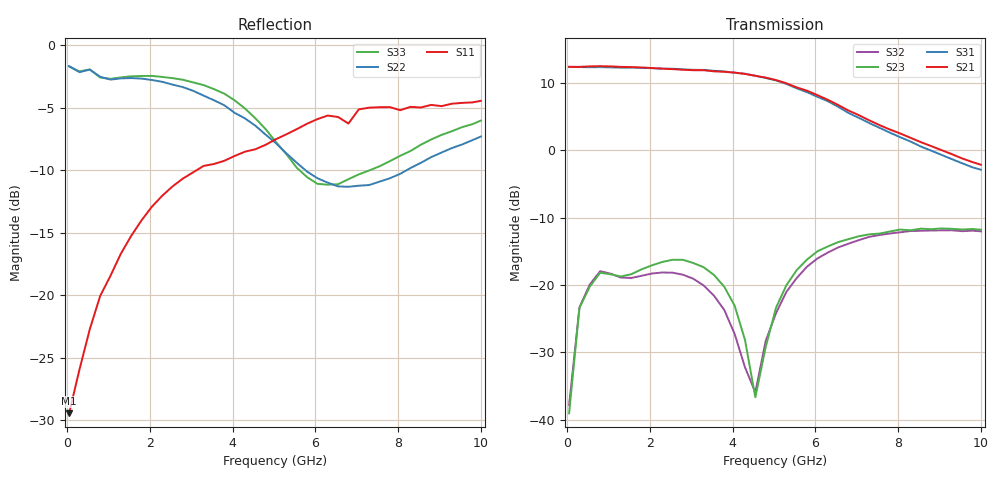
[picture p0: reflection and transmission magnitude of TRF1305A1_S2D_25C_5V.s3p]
! Created Tue Jun 24 15:00:24 2025
# hz S ma R 50
! 3 Port Network Data from SP1.SP block
! PORT[1] = INP
! PORT[2] = OUTM
! PORT[3] = OUTP
! freq  magS11  angS11  magS12  angS12  magS13  angS13
!  magS21  angS21
!  magS22  angS22  magS23  angS23
!  magS31  angS31  magS32  angS32
!  magS33  angS33
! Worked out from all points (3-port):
!   41 points, 50 MHz to 10 GHz, reference 50 ohm
!   strongest paths, dB at 50 MHz, 2.55 GHz, 5.05 GHz, 7.55 GHz, 10 GHz:
!     S21: 12.4, 12.0, 10.4, 3.7, -2.2
!     S31: 12.3, 12.1, 10.3, 3.3, -2.9
!     S23: -39.0, -16.2, -23.4, -12.4, -11.8
!     S32: -37.8, -18.2, -24.2, -12.6, -12.0
!   lowest |S11| = -29.5 dB at 50 MHz (marker M1), VSWR 1.07, Z = 46.8 - j0.755 ohm
!   |S11| at or under -10 dB: start of sweep to 3.132 GHz
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5e7  0.03365 -166.2  0.003272 -15.6  0.003012 154.3
     4.154 178.6  0.8248 178.5  0.0112 138.5
     4.14 -1.5  0.01293 124.3  0.8229 178.1
3e8  0.05036 -135.1  0.01217 51.3  0.008879 56.0
     4.146 170.9  0.7803 170.7  0.06782 55.6
     4.137 -9.5  0.06833 53.7  0.7863 171.0
1.05e9  0.1196 -108.7  0.03335 47.6  0.022 46.4
        4.184 146.9  0.7287 156.0  0.1202 24.9
        4.114 -32.0  0.1216 20.0  0.7341 157.4
2.55e9  0.2724 -103.2  0.05602 28.8  0.0305 13.5
        3.992 99.9  0.6961 123.5  0.154 0.9
        4.017 -78.6  0.1236 -2.5  0.7386 126.3
3.8e9  0.3448 -103.9  0.07248 8.5  0.03515 -15.7
       3.816 59.1  0.5754 96.8  0.09707 -46.5
       3.832 -120.1  0.06528 -31.8  0.6403 97.3
4.55e9  0.3835 -102.9  0.07964 -5.8  0.03309 -35.1
        3.561 31.9  0.4765 83.6  0.01472 -147.0
        3.565 -147.9  0.01603 44.3  0.5102 81.0
5.05e9  0.421 -100.4  0.08114 -14.7  0.02872 -46.6
        3.312 13.4  0.4052 77.8  0.06798 105.3
        3.291 -166.8  0.06197 83.2  0.4098 74.7
6.55e9  0.5162 -109.8  0.08132 -40.8  0.02081 -50.7
        2.164 -36.7  0.2724 83.2  0.2081 48.6
        2.1 141.4  0.19 49.7  0.2779 91.9
8.3e9  0.5668 -121.3  0.06898 -66.0  0.01443 -88.2
       1.236 -75.5  0.3227 92.5  0.2546 14.4
       1.16 100.7  0.2515 17.1  0.3775 97.3
1e10  0.5994 -134.5  0.05453 -85.9  0.01027 -129.1
      0.7804 -105.4  0.4312 82.0  0.2572 -7.4
      0.7163 69.3  0.2502 -6.8  0.4995 85.9
